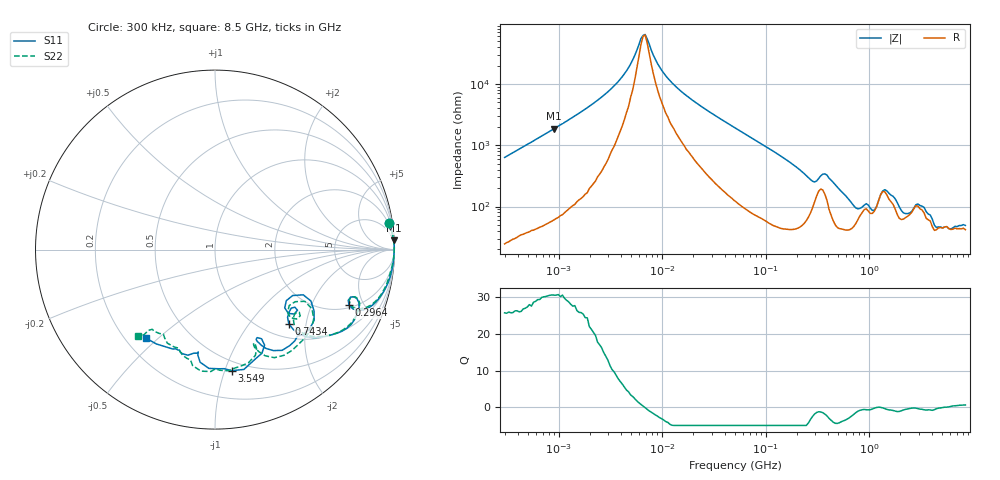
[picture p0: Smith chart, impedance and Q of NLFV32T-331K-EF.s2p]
! S-parameter Generated by TDK Corporation
! Copyright(C) 2015 TDK Corporation.
! All Rights Reserved.
! TDK P/N: NLFV32T-331K-EF (Inductors)
! Property: L=330uH at 796kHz
! Size(LxWxT): 3.2x2.5x2.2mm, 0.126x0.098x0.087inches
! Model Type: s2p (Touchstone File Format Version 1.0)
! Frequency: DC=Yes Start=0.3MHz Stop=8500MHz 225points Log-sweep
! Note:
! Model Generated on Jun. 23, 2015
! Hash(MD5):
! Port Assignments:
!  1 ---@@@--- 2
! Applicable Conditions:
!  Temperature = 25 degC
!  DC Bias Current = 0 A
!  Small Signal Operation
! Terms and conditions regarding TDK Simulation Models
! (1)This simulation model is being provided solely for informational purposes. Please refer to the specifications of the products in terms of detailed characteristics of such products.
! (2)In no event shall TDK Corporation of any of its subsidiaries be liable for any loss or damage arising, directly or indirectly,
!  From any information contained in this simulation model, including, but not limited to loss or damages arising from any inaccuracies, omissions or errors in connection with such information.
! (3)Any and all copyrights on this simulation model are owned by TDK Corporation.
!  Duplication or redistribution of this simulation model without prior written permission from TDK Corporation is prohibited.
! (4)This simulation model is subject to any modification or change without any prior notice.
! (5)Neither TDK Corporation nor any of its subsidiaries shall make any warranty, express or implied,
!  Including but not limited to the correctness, implied warranties of merchantability and fitness for a particular purpose with respect to this simulation models.
! (6)The use of this simulation model shall be deemed to have consented to the terms and conditions hereof.
# MHz S MA R 50
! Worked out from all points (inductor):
!   224 points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, 300 kHz to 8.5 GHz, reference 50 ohm
!   read as one part in series: L = 332 uH near 314.1 kHz
!   highest Q = 30.6 at 904.3 kHz (marker M1), where L = 328 uH
!   self-resonance near 6.528 MHz
!   S11 on the Smith chart (normalised r, x): 300 kHz: 2, +13; 296.4 MHz: 2.15, -3.87; 743.4 MHz: 1.28, -1.60; 3.549 GHz: 0.42, -1.06; 8.5 GHz: 0.28, -0.46
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0.3  0.9822 8.6  0.1553 -79.2  0.1573 -79.4  0.9815 8.6
0.9042579  0.9965 2.9  0.0534 -85.2  0.05367 -85.6  0.9965 2.9
1.72111  0.9983 1.4  0.02707 -86.3  0.02716 -86.7  0.9989 1.4
3.937196  0.9988 0.4  0.008313 -81.6  0.008332 -82.0  0.9988 0.2
6.528405  0.9985 -0.1  0.001611 -14.8  0.001607 -15.5  0.9983 -0.3
9.430415  0.9982 -0.5  0.005273 70.2  0.005281 69.8  0.9982 -0.6
16.37255  0.9979 -1.2  0.01454 80.6  0.01454 80.3  0.9977 -1.3
51.67171  0.996 -4.1  0.0529 82.2  0.05293 82.0  0.9934 -4.2
170.7477  0.9681 -14.0  0.1814 71.5  0.1815 71.3  0.9647 -13.9
283.1228  0.8374 -23.3  0.3167 46.0  0.317 45.8  0.8366 -22.8
296.4424  0.8092 -22.6  0.3154 40.3  0.3156 40.0  0.8109 -22.1
373.0505  0.8548 -20.3  0.2464 42.6  0.2466 42.3  0.8582 -20.2
564.2308  0.7813 -38.2  0.4475 38.3  0.4475 38.1  0.7906 -37.2
743.4462  0.5828 -45.1  0.5517 16.0  0.5517 15.7  0.6074 -43.5
1232.735  0.5523 -27.1  0.4255 -19.1  0.426 -19.4  0.577 -30.0
1551.304  0.6815 -44.2  0.3565 -1.4  0.3569 -2.0  0.7026 -46.0
2044.041  0.6201 -62.7  0.4956 -7.6  0.4962 -7.8  0.6184 -66.8
2693.286  0.5605 -62.4  0.4399 -31.6  0.4401 -32.2  0.5985 -67.2
3548.748  0.6808 -82.2  0.4235 -27.3  0.4244 -27.8  0.6731 -87.5
4265.177  0.633 -97.5  0.4895 -36.0  0.4894 -36.0  0.658 -100.9
6161.135  0.6037 -108.6  0.4621 -67.4  0.4579 -67.6  0.5659 -119.8
8500  0.6257 -128.0  0.336 -101.9  0.3357 -101.1  0.6434 -131.6
